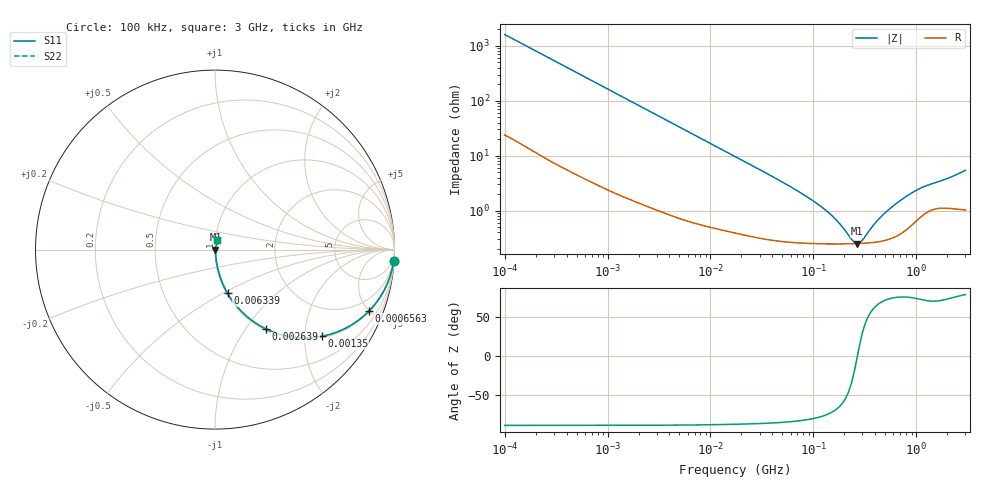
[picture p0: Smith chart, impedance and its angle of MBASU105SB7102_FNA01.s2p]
! MBASU105SB7102_FNA01  S-PARAMETER MODEL  ( Standard Model )
! Model Generated by TAIYO YUDEN Corporation (http://www.ty-top.com)
! Version 1.0
! TAIYO YUDEN Control No. 220601
! Copyright(c) 2013 TAIYO YUDEN CO.,LTD. All Rights Reserved.
! Product Description (link to TY-COMPAS)
! https://ds.yuden.co.jp/TYCOMPAS/or/detail?pn=MBASU105SB7102KFNA01&u=M
! Products Name : Multilayer Ceramic Capacitors
! Characteristics :
!  Capacitance : 1000 [pF] , Rated Voltage : 50 [V] , TCC : X7R
!  Case Size : 1.0 x 0.5 / 0.039 x 0.02 [mm/inch] , Thickness : 0.5 / 0.02 [mm/inch]
!  (Conditions: Temperature = 25 [degC] , DC Bias Voltage = 0 [V])
! External Node Assignments :
!  1  o---| |---o  2
! GND o---------o GND
! Frequency Range : 100kHz  -  3GHz  [ 401 STEP ]
# MHZ S RI R 50
! Freq[MHz].  S11 Real  S11 Imag  S21 Real  S21 Imag  S12 Real  S12 Imag  S22 Real  S22 Imag
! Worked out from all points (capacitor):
!   401 points, 100 kHz to 3 GHz, reference 50 ohm
!   read as one part in series: C = 986 pF near 105.3 kHz
!   lowest |Z| = 251 mohm at 266.1 MHz (marker M1)
!   series resonance near 267.9 MHz, so ESL is about 360 pH
!   S11 on the Smith chart (normalised r, x): 100 kHz: 1, -32; 656.3 kHz: 1.07, -4.99; 1.35 MHz: 1.04, -2.44; 2.639 MHz: 1.02, -1.25; 6.339 MHz: 1.01, -0.53; 3 GHz: 1.02, +0.11
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0.1  0.9952 -0.0618  0.00476 0.0618  0.00476 0.0618  0.9952 -0.0618
0.246461  0.9755 -0.1478  0.0245 0.1478  0.0245 0.1478  0.9755 -0.1478
0.562235  0.8908 -0.305  0.1092 0.305  0.1092 0.305  0.8908 -0.305
0.656258  0.858 -0.3422  0.142 0.3422  0.142 0.3422  0.858 -0.3422
0.941399  0.7492 -0.4263  0.2508 0.4263  0.2508 0.4263  0.7492 -0.4263
1.350433  0.5961 -0.4831  0.4039 0.4831  0.4039 0.4831  0.5961 -0.4831
1.887902  0.4341 -0.4875  0.5659 0.4875  0.5659 0.4875  0.4341 -0.4875
2.639283  0.2856 -0.4429  0.7144 0.4429  0.7144 0.4429  0.2856 -0.4429
3.161081  0.22 -0.405  0.78 0.405  0.78 0.405  0.22 -0.405
6.3393  0.0697 -0.2431  0.9303 0.2431  0.9303 0.2431  0.0697 -0.2431
17.7727  0.0126 -0.093  0.9874 0.093  0.9874 0.093  0.0126 -0.093
51.12795  0.00373 -0.0319  0.9963 0.0319  0.9963 0.0319  0.00373 -0.0319
97.38194  0.00274 -0.0152  0.9973 0.0152  0.9973 0.0152  0.00274 -0.0152
154.8634  0.00252 -0.00733  0.9975 0.00733  0.9975 0.00733  0.00252 -0.00733
240.0085  0.00249 -0.00141  0.9975 0.00141  0.9975 0.00141  0.00249 -0.00141
266.0711  0.0025 -8.79e-05  0.9975 8.79e-05  0.9975 8.79e-05  0.0025 -8.79e-05
294.964  0.00253 0.00124  0.9975 -0.00124  0.9975 -0.00124  0.00253 0.00124
412.3589  0.0027 0.00575  0.9973 -0.00575  0.9973 -0.00575  0.0027 0.00575
547.5153  0.00311 0.0102  0.9969 -0.0102  0.9969 -0.0102  0.00311 0.0102
765.4251  0.00444 0.0165  0.9956 -0.0165  0.9956 -0.0165  0.00444 0.0165
1042.837  0.00742 0.023  0.9926 -0.023  0.9926 -0.023  0.00742 0.023
3000  0.0129 0.0519  0.9871 -0.0519  0.9871 -0.0519  0.0129 0.0519
